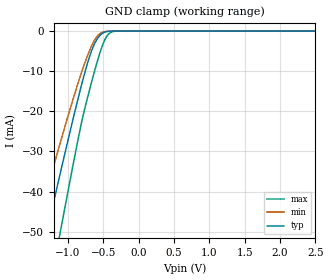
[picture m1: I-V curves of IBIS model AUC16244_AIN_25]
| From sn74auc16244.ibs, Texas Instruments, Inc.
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[Model]   AUC16244_AIN_25
Model_type  Input
Vinl=0.7
Vinh=1.7
| variable   typ   min   max
C_comp   3.21pF   2.44pF   3.75pF
[Temperature Range]   40   100   -40
| Ambient temperature   25   85   -40
[Voltage range]   2.5   2.3   2.7
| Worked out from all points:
|   GND clamp passes 1 mA (typ) near -0.54 V on its own axis
[GND Clamp]
| AUC16244_AIN_25
|   Voltage   I(typ)   I(min)   I(max)
-3.6V     -231.9mA   -193.8mA   -279.4mA
-1.485V   -64.54mA   -51.6mA    -85.16mA
-1.435V   -60.63mA   -48.38mA   -80.51mA
-1.3V     -50.12mA   -39.75mA   -67.93mA
-1.115V   -35.9mA    -28.19mA   -50.67mA
-830mV    -14.93mA   -11.49mA   -24.63mA
-720mV    -7.795mA   -5.96mA    -16.35mA
-625mV    -3.211mA   -2.297mA   -10.05mA
-525mV    -720.2uA   -383.4uA   -4.21mA
-430mV    -77.57uA   -37uA      -820.2uA
-325mV    -3.541uA   -2.134uA   -32.63uA
2.5V      338.1pA    432.6pA    502.6pA
